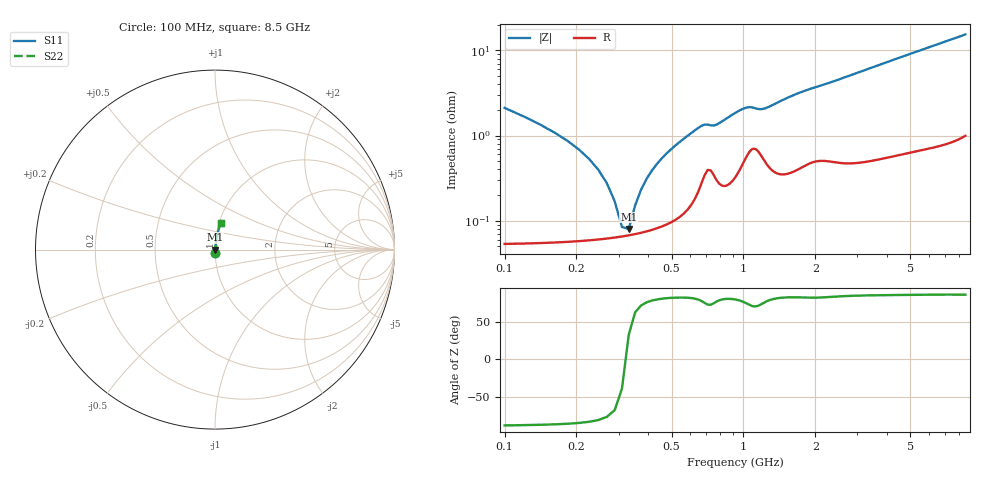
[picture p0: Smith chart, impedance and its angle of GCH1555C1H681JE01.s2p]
!Murata Part Number: GCH1555C1H681JE01
!These Parameters are Measured in Series Mode Connection
!Data Generated on Jun 19, 2026
!  o--ll--o
!Port1  Port2
!  o------o
!Operation Temp=25[degC], DC Bias Voltage=0[V]
!Freq. Start=100[MHz] Stop=9[GHz] 401[Steps]
# Hz S RI R 50
!Freq.(Hz) S11(Real) S11(Imag) S21(Real) S21(Imag) S12(Real) S12(Imag) S22(Real) S22(Imag)
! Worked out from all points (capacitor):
!   401 points, 100 MHz to 8.5 GHz, reference 50 ohm
!   read as one part in series: C = 678 pF near 142 MHz
!   lowest |Z| = 79.9 mohm at 331 MHz (marker M1)
!   series resonance near 321.6 MHz, so ESL is about 360 pH
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1e8  0.000979 -0.0211  0.999 0.0211  0.999 0.0211  0.000979 -0.0211
1.42e8  0.000722 -0.0133  0.9993 0.0133  0.9993 0.0133  0.000722 -0.0133
2.05e8  0.00062 -0.0068  0.9994 0.0068  0.9994 0.0068  0.00062 -0.0068
2.47e8  0.000615 -0.0039  0.9994 0.0039  0.9994 0.0039  0.000615 -0.0039
2.89e8  0.000635 -0.00157  0.9994 0.00157  0.9994 0.00157  0.000635 -0.00157
3.1e8  0.000651 -0.000534  0.9993 0.000534  0.9993 0.000534  0.000651 -0.000534
3.31e8  0.000672 0.000431  0.9993 -0.000431  0.9993 -0.000431  0.000672 0.000431
3.52e8  0.000696 0.00134  0.9993 -0.00134  0.9993 -0.00134  0.000696 0.00134
4.15e8  0.000795 0.00384  0.9992 -0.00384  0.9992 -0.00384  0.000795 0.00384
4.57e8  0.000886 0.00538  0.9991 -0.00538  0.9991 -0.00538  0.000886 0.00538
5.41e8  0.00117 0.00833  0.9988 -0.00833  0.9988 -0.00833  0.00117 0.00833
6.46e8  0.00231 0.012  0.9977 -0.012  0.9977 -0.012  0.00231 0.012
7.72e8  0.00315 0.013  0.9968 -0.013  0.9968 -0.013  0.00315 0.013
1.003e9  0.00527 0.02  0.9947 -0.02  0.9947 -0.02  0.00527 0.02
1.213e9  0.00563 0.0197  0.9944 -0.0197  0.9944 -0.0197  0.00563 0.0197
1.507e9  0.00423 0.0269  0.9958 -0.0269  0.9958 -0.0269  0.00423 0.0269
1.927e9  0.00601 0.0351  0.994 -0.0351  0.994 -0.0351  0.00601 0.0351
2.914e9  0.00747 0.0524  0.9925 -0.0524  0.9925 -0.0524  0.00747 0.0524
4.3e9  0.0117 0.0772  0.9883 -0.0772  0.9883 -0.0772  0.0117 0.0772
5.707e9  0.0172 0.1013  0.9828 -0.1013  0.9828 -0.1013  0.0172 0.1013
7.114e9  0.0239 0.125  0.9761 -0.125  0.9761 -0.125  0.0239 0.125
8.5e9  0.0323 0.1475  0.9677 -0.1475  0.9677 -0.1475  0.0323 0.1475
